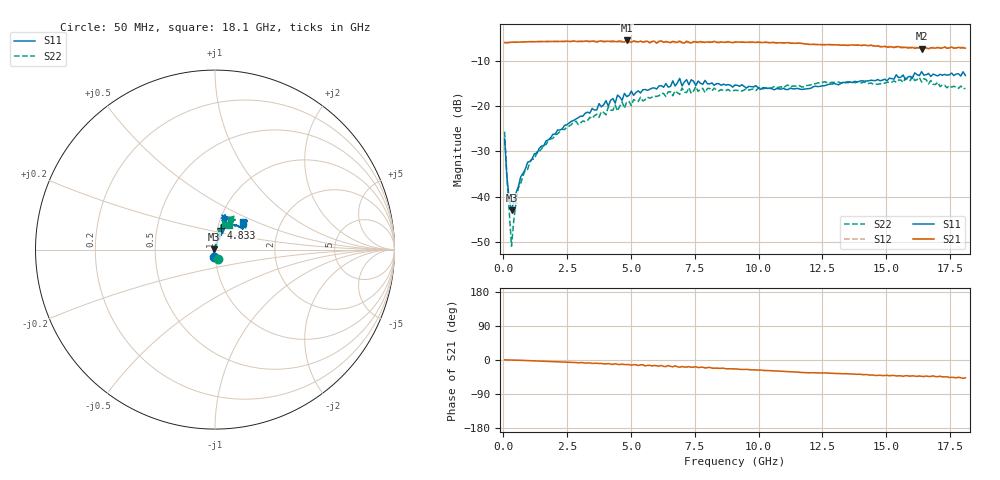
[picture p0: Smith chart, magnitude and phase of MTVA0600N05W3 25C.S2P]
! Network Analyzer HP8720D.06.14 Serial No. US36140669
!  8 Jul 2005  13:14:10
! Frequency  S11  S21  S12  S22
# HZ  S  DB R 50
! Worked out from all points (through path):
!   201 points, 50 MHz to 18.1 GHz, reference 50 ohm
!   highest |S21| = -5.47 dB at 4.833 GHz (marker M1); lowest = -7.3 dB at 16.39 GHz (marker M2)
!   group delay of S21, straight-line fit = 7.6 ps
!   lowest |S11| = -43.0 dB at 320.8 MHz (marker M3), VSWR 1.01, Z = 49.3 + j0.162 ohm
!   |S11| at or under -10 dB: start of sweep to end of sweep
!   |S22| runs from -51.0 to -13.4 dB; largest |S21 - S12| = 0.025
!   S11 on the Smith chart (normalised r, x): 50 MHz: 0.99, -0.09; 4.833 GHz: 1.04, +0.26; 18.1 GHz: 1.29, +0.42
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5e7  -27.17 -96.6  -5.93 0.4  -5.92 0.4  -25.66 -73.4
1.4025e8  -35.57 -116.8  -5.97 0.2  -5.95 0.2  -35.89 -101.3
2.305e8  -40.73 -147.1  -5.92 0.2  -5.88 0.1  -43.23 -123.3
3.2075e8  -43.04 166.6  -5.86 0.2  -5.87 0.2  -50.97 163.5
4.11e8  -41.04 130.1  -5.87 -0.3  -5.85 -0.3  -45.13 112.8
5.915e8  -37.73 104.7  -5.81 -0.4  -5.83 -0.5  -38.05 93.1
1.04275e9  -32.22 86.2  -5.74 -1.8  -5.73 -1.7  -32.31 77.2
2.12575e9  -25.28 69.7  -5.68 -4.8  -5.67 -4.7  -26.09 73.9
3.1185e9  -22.22 70.7  -5.68 -7.0  -5.71 -7.4  -23.29 79.0
4.47225e9  -17.54 65.5  -5.76 -11.4  -5.61 -10.5  -21.07 81.2
4.83325e9  -17.89 74.6  -5.47 -12.0  -5.69 -12.8  -19.05 70.8
6.09675e9  -15.54 69.7  -5.70 -16.0  -5.62 -15.8  -17.70 73.8
6.7285e9  -15.55 76.4  -5.77 -15.5  -6.01 -16.5  -16.63 69.5
6.909e9  -13.86 74.1  -5.60 -19.1  -5.73 -17.5  -17.40 68.7
6.99925e9  -15.53 74.1  -5.90 -17.2  -6.02 -19.1  -15.97 70.2
7.17975e9  -14.13 78.6  -5.63 -18.5  -5.89 -17.5  -16.99 65.6
9.075e9  -15.32 73.0  -5.82 -23.6  -5.80 -23.7  -16.49 65.1
1.21435e10  -15.70 55.7  -6.34 -33.5  -6.30 -33.6  -15.17 61.8
1.512175e10  -13.82 37.6  -6.94 -41.7  -6.76 -41.2  -14.77 65.7
1.602425e10  -13.87 42.5  -7.00 -41.5  -7.18 -43.9  -13.42 60.6
1.638525e10  -12.38 42.0  -7.32 -43.1  -7.10 -42.2  -14.67 60.0
1.81e10  -13.22 44.8  -7.17 -46.9  -7.37 -47.7  -16.07 60.7
